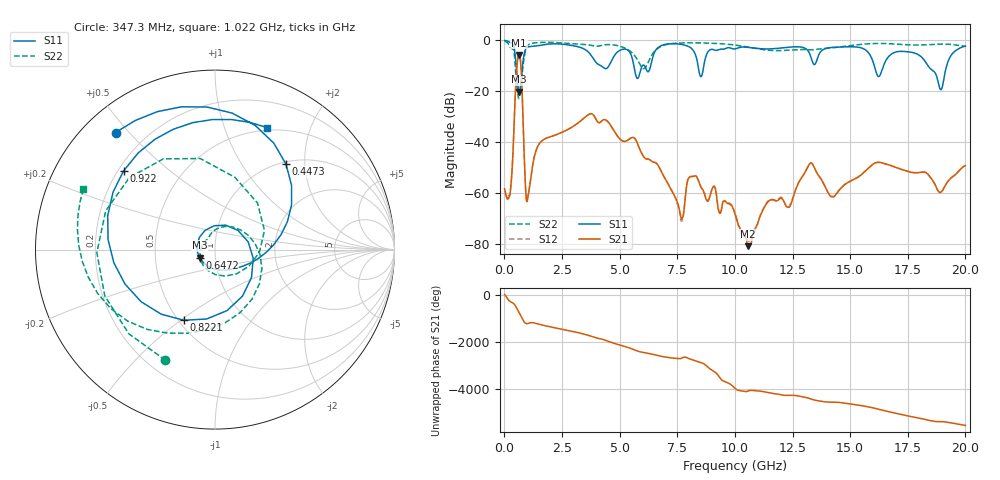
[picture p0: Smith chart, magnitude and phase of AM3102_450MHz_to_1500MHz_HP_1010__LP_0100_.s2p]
!Agilent Technologies,E8364B,MY43040894,A.07.50.67
!Agilent E8364B: A.07.50.67
!Date: Thursday, January 11, 2018 06:10:54
!Correction: S11(Full 2 Port(1,2))
!S21(Full 2 Port(1,2))
!S12(Full 2 Port(1,2))
!S22(Full 2 Port(1,2))
!S2P File: Measurements: S11, S21, S12, S22:
# Hz S  dB  R 50
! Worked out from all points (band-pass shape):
!   1601 points, 10 MHz to 20 GHz, reference 50 ohm
!   highest |S21| = -5.79 dB at 634.7 MHz (marker M1); lowest = -81.0 dB at 10.57 GHz (marker M2)
!   |S21| within 3 dB of the highest: 559 MHz to 707.4 MHz (148.5 MHz wide, 23.4 % of centre)
!   lowest |S11| = -20.3 dB at 647.2 MHz (marker M3), VSWR 1.21, Z = 41.9 - j3.75 ohm
!   |S11| at or under -10 dB: 5.617 GHz to 5.989 GHz (371.6 MHz wide, 6.4 % of centre); 16.05 GHz to 16.45 GHz (400.3 MHz wide, 2.46 % of centre); 18.38 GHz to 19.19 GHz (811.3 MHz wide, 4.32 % of centre)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
!   |S22| runs from -23.0 to -0.3 dB; largest |S21 - S12| = 0.0013
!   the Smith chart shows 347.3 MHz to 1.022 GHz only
!   S11 on the Smith chart (normalised r, x): 347.3 MHz: 0.09, +0.46; 447.3 MHz: 1.04, +1.61; 647.2 MHz: 0.84, -0.07; 822.1 MHz: 0.53, -0.51; 922 MHz: 0.22, +0.35; 1.022 GHz: 0.47, +1.41
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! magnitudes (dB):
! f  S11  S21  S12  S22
! 10 MHz  -0.1  -58.5  -59.4  -0.3
! 347.3 MHz  -1.4  -49.0  -49.0  -3.4
! 447.3 MHz  -4.2  -27.0  -27.0  -7.6
! 634.7 MHz  -20.2  -5.8  -5.8  -23.0
! 647.2 MHz  -20.3  -5.9  -5.9  -22.5
! 822.1 MHz  -7.3  -35.3  -35.3  -9.3
! 922 MHz  -3.5  -58.8  -58.7  -3.5
! 1.022 GHz  -2.6  -61.6  -61.2  -1.9
! 1.534 GHz  -2.0  -40.5  -40.5  -0.9
! 3.346 GHz  -3.0  -31.4  -31.4  -1.5
! 5.782 GHz  -15.0  -40.8  -40.8  -7.8
! 6.682 GHz  -2.8  -49.4  -49.4  -3.0
! 7.681 GHz  -1.6  -70.5  -71.2  -1.0
! 8.193 GHz  -4.0  -53.6  -53.6  -1.0
! 8.531 GHz  -14.3  -57.9  -57.7  -1.0
! 10.01 GHz  -3.4  -68.5  -68.0  -1.9
! 10.57 GHz  -2.8  -81.0  -78.7  -2.7
! 13.34 GHz  -7.8  -48.4  -48.5  -3.8
! 14.23 GHz  -2.8  -61.5  -61.6  -3.0
! 16.68 GHz  -6.3  -49.0  -49.0  -1.3
! 18.94 GHz  -19.4  -59.8  -59.8  -1.5
! 20 GHz  -2.3  -49.4  -49.2  -2.4
